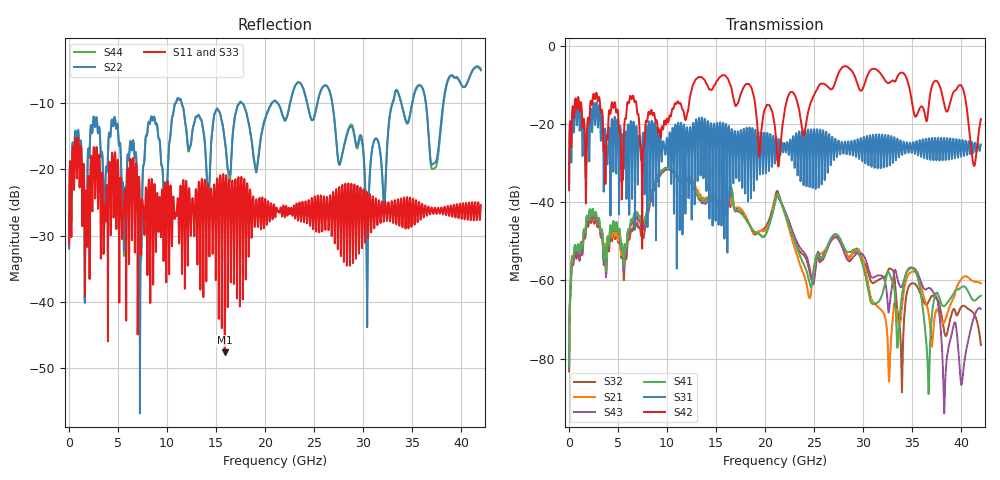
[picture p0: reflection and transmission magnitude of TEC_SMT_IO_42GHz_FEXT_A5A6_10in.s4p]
!! CHANNEL DESCRIPTION: Next Generation 28Gbps High Density SMT I/O Connector
!!  with 10" 5-6-5 Megatron 6 Stripline trace on host side and 1.25" 7-5-7 Megtron 6 Microstrip trace on plug side at 14GHz
!! HOST PCB DESCRIPTION: PCB thickness 2.86 mm, Nelco 4000-13SI (Dk 3.32, Df 0.010)
!!  23 Layer Board, 12 GND planes, 2 Layer route-out on Layers 10,12, 8 mil stub on vias
!!  Pairs on following layers
!!  Layer 12 - A5A6
!! CONNECTOR DESCRIPTION:  Next Generation 28Gbps High Density SMT I/O Connector
!! PLUG-IN CARD DESCRIPTION:  PCB thickness 1mm thick, Nelco 4000-13SI (Dk 3.32, Df 0.010)
!!  6 Layer Board, 4 GND planes, 0.35 x 1.4mm mating pads
!!  Micro-strip diff traces referenced to GND plane 3mils down, 2nd GND plane 15mils from top of board
!!  PCB GND planes are symmetric
!! MODEL DESCRIPTION: TE Connectivity S-parameter model produced from Macro-model
!! MODEL DATE: 9/25/2014 CR1a_GC1i, VR6&12_4
!! MODEL STATUS: Developmental
!! MODEL GEOMETRY: 2 Rows - Rows A, B. 3 pairs in each row, 6 total pairs
!! MODEL FREQUENCY RANGE: DC to 42 GHz in 10 MHz frequency steps
!! MODEL EDGE RATE LIMITATION: 11.90 ps (Using conservative 0.5/Fmax rule of thumb)
!! TIME-DOMAIN TRANSFORM CAUTIONS:
!! 1.) Do not simulate transient edge rates faster than the number listed above.  Edge
!!  rates faster than this number contain significant spectral content at frequencies
!!  above the model's highest frequency.
!! 2.) Even when simulating edge rates that are slower than the number listed above, be
!!  aware that the best time resolution possible with a direct iFFT is (1 / 2Fmax).
!!  As a result, time resolution is typically not adequate for most time-domain
!!  simulations unless tricks such as frequency-domain zero-padding and windowing are
!!  used to minimize leakage and aliasing.
!! 3.) Because the model has a uniform frequency step, a direct iFFT will result in an
!!  impulse that that has a time length given by either (1 / Fstep) or (1 / 2Fstep),
!!  depending on the transform being used.  Care has been taken in selecting the
!!  frequency step to ensure a settled impulse response for the model.  Therefore,
!!  convolution with the model's impulse response should present no issues.  However,
!!  if directly concatenating s-parameter models in the frequency domain a user must
!!  either interpolate necessary interim frequencies or complete impulse response
!!  zero-padding.  Impulse response zero-padding is more difficult, but more accurate.
!! PORT DEFINITIONS:
!! Port  1  ----->  Host, Bot Row  A5  B5  Module, Top Row  <-----  Port  2
!! Port  3  ----->  Host, Bot Row  A6  B6  Module, Top Row  <-----  Port  4
# Hz S MA R 50
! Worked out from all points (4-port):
!   4200 points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, 10 MHz to 42 GHz, reference 50 ohm
!   strongest paths, dB at 10 MHz, 10.51 GHz, 21.01 GHz, 31.51 GHz, 42 GHz:
!     S42: -36.7, -16.2, -21.0, -6.3, -18.7
!     S31: -36.9, -22.4, -28.6, -27.9, -25.2
!     S41: -81.9, -31.8, -39.9, -65.6, -63.9
!     S43: -82.6, -32.2, -39.9, -58.7, -67.3
!     S21: -82.5, -31.6, -39.1, -66.7, -60.7
!     S32: -83.3, -31.8, -38.6, -59.9, -76.5
!   lowest |S11| = -47.6 dB at 15.88 GHz (marker M1), VSWR 1.01, Z = 50.4 + j0.0744 ohm
!   |S11| at or under -10 dB: start of sweep to end of sweep
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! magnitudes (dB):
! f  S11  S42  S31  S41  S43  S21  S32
! 10 MHz  -31.3  -36.7  -36.9  -81.9  -82.6  -82.5  -83.3
! 2.25 GHz  -17.9  -14.0  -16.3  -43.5  -44.1  -44.3  -45.2
! 15.88 GHz  -47.6  -7.5  -30.4  -41.0  -42.3  -40.6  -40.6
! 21.36 GHz  -26.4  -30.8  -24.4  -37.9  -38.9  -38.1  -37.9
! 32.66 GHz  -26.2  -9.4  -27.2  -58.1  -67.0  -85.2  -56.9
! 36.62 GHz  -25.7  -16.8  -25.1  -85.1  -61.9  -67.7  -65.7
! 42 GHz  -25.4  -18.7  -25.2  -63.9  -67.3  -60.7  -76.5
